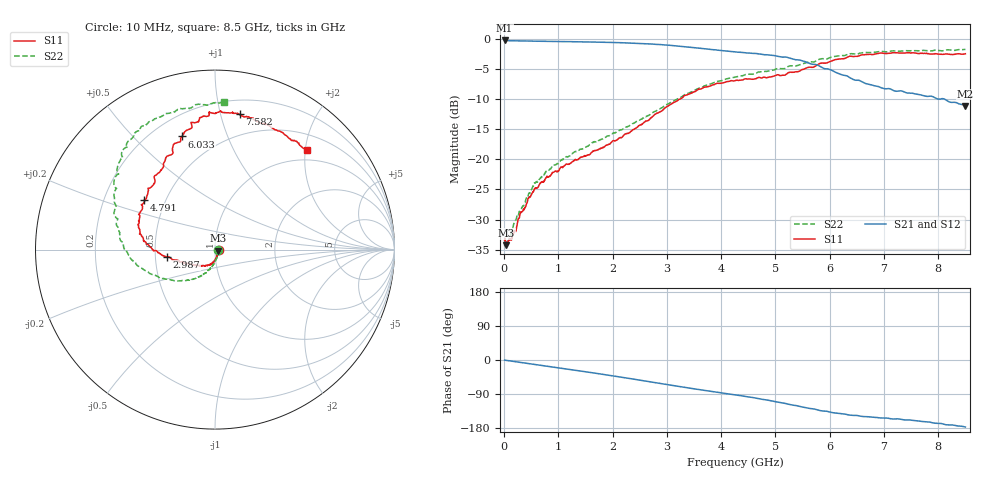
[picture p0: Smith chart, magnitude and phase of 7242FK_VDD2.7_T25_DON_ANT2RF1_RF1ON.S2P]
!Agilent Technologies,E5071C,MY46417908,A.11.23
!Date: Wed Dec 09 15:38:46 2020
!Data & Calibration Information:
!Freq	S11:SOLT2(ON)	S21:SOLT2(ON)	S12:SOLT2(ON)	S22:SOLT2(ON)
!PortZ  Port1:50+j0  Port2:50+j0
!Above PortZ is port z conversion or system Z0 setting when saving the data.
!When reading, reference impedance value at option line is always used.
# Hz S dB R 50
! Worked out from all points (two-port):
!   1601 points, 10 MHz to 8.5 GHz, reference 50 ohm
!   highest |S21| = -0.22 dB at 10 MHz (marker M1); lowest = -11.1 dB at 8.5 GHz (marker M2)
!   |S21| within 3 dB of the highest: start of sweep to 5.284 GHz
!   lowest |S11| = -34.3 dB at 41.84 MHz (marker M3), VSWR 1.04, Z = 51.9 - j0.639 ohm
!   |S11| at or under -10 dB: start of sweep to 3.228 GHz
!   |S22| runs from -34.4 to -1.7 dB; largest |S21 - S12| = 0.0038
!   S11 on the Smith chart (normalised r, x): 10 MHz: 1.04, -0.00; 2.987 GHz: 0.57, -0.05; 4.791 GHz: 0.38, +0.28; 6.033 GHz: 0.32, +0.70; 7.582 GHz: 0.31, +1.15; 8.5 GHz: 0.79, +2.04
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1e7  -33.48 -2.9  -0.22 -0.3  -0.23 -0.3  -34.43 -10.7
4.18375e7  -34.31 -18.7  -0.25 -1.0  -0.25 -1.0  -33.84 -19.1
9.49e7  -33.48 -34.6  -0.27 -2.1  -0.26 -2.1  -33.21 -36.5
1.744938e8  -32.35 -52.2  -0.27 -3.8  -0.28 -3.8  -30.88 -50.7
2.965375e8  -28.99 -70.6  -0.29 -6.3  -0.30 -6.3  -28.65 -68.8
5.671562e8  -24.83 -88.5  -0.35 -11.8  -0.35 -11.8  -23.92 -88.2
9.120625e8  -22.17 -100.4  -0.39 -18.8  -0.39 -18.8  -21.11 -97.7
1.426769e9  -19.59 -120.4  -0.46 -29.5  -0.46 -29.5  -18.29 -108.5
2.079438e9  -16.80 -144.4  -0.59 -43.5  -0.59 -43.5  -15.38 -118.8
2.843538e9  -12.24 -166.9  -0.89 -61.1  -0.90 -61.1  -11.68 -138.1
2.986806e9  -11.30 -171.3  -0.99 -64.4  -0.99 -64.4  -10.91 -142.1
3.586412e9  -8.33 175.6  -1.51 -77.9  -1.51 -77.9  -8.17 -160.5
4.255e9  -6.91 159.5  -2.12 -92.0  -2.12 -92.0  -6.32 -176.5
4.790931e9  -6.34 144.7  -2.59 -104.5  -2.57 -104.5  -5.39 170.8
5.194206e9  -5.88 131.2  -2.98 -115.0  -2.96 -115.1  -4.79 162.3
5.671769e9  -4.70 115.3  -4.17 -128.5  -4.13 -128.5  -3.79 148.4
6.032594e9  -3.65 106.3  -5.17 -138.4  -5.19 -138.1  -2.99 140.2
6.41995e9  -2.88 99.6  -6.63 -146.0  -6.66 -145.7  -2.42 131.6
7.088538e9  -2.37 89.6  -8.23 -154.1  -8.26 -154.3  -2.07 122.1
7.582019e9  -2.31 79.7  -9.12 -160.2  -9.14 -160.0  -1.91 113.4
7.911006e9  -2.47 68.8  -9.61 -166.3  -9.62 -166.3  -1.88 105.6
8.5e9  -2.44 47.1  -11.14 -176.8  -11.21 -176.7  -1.70 86.4
